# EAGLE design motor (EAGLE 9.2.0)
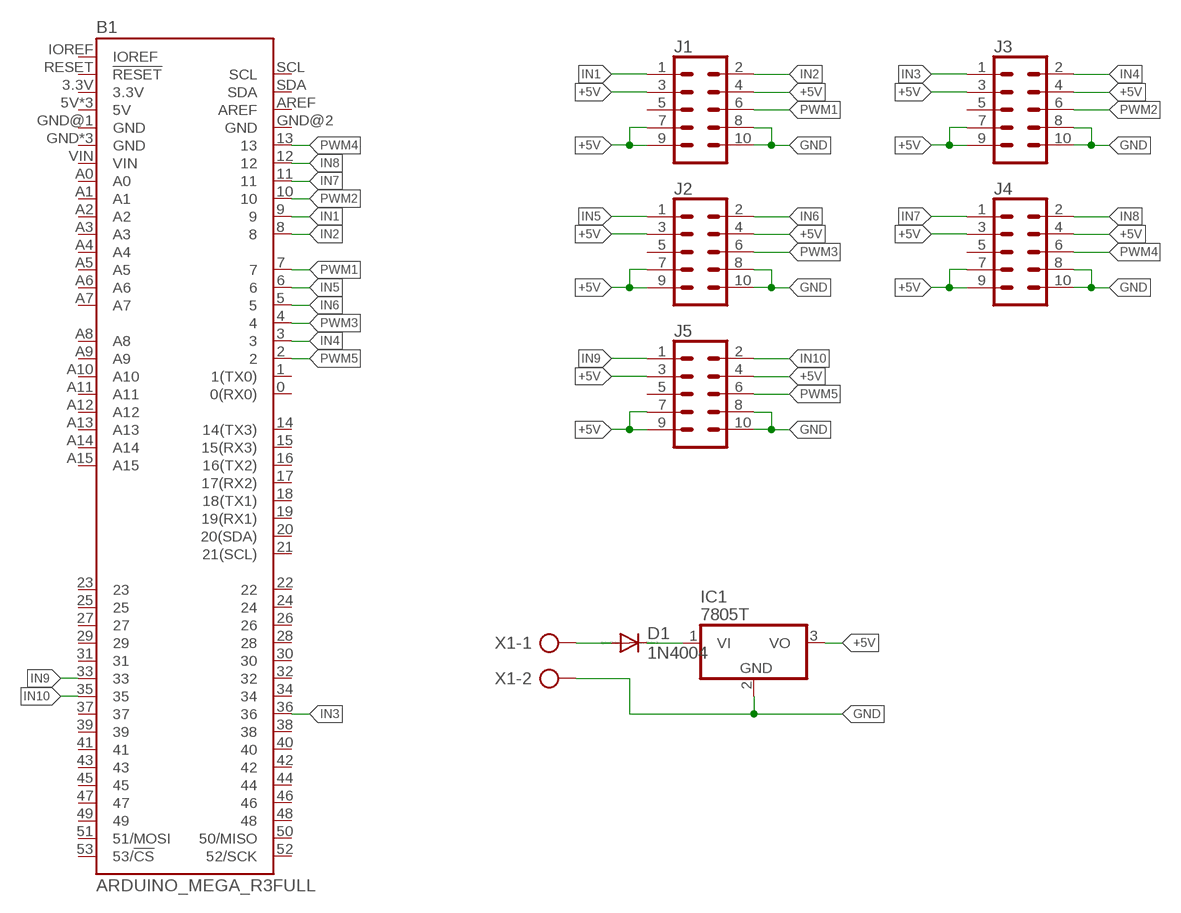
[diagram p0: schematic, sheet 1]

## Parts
B1  ARDUINO_MEGA_R3FULL  [ARDUINO_MEGA_NO_SILK]
D1  1N4004  [DO41-10]
IC1  7805T  [TO220H]
J1  CONN_05X2SHD-NS  [2X5-SHROUDED-NS]
J2  CONN_05X2SHD-NS  [2X5-SHROUDED-NS]
J3  CONN_05X2SHD-NS  [2X5-SHROUDED-NS]
J4  CONN_05X2SHD-NS  [2X5-SHROUDED-NS]
J5  CONN_05X2SHD-NS  [2X5-SHROUDED-NS]
X1  AK300/2  [AK300/2]

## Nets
+5V: IC1.3(VO) J1.3 J1.4 J1.7 J1.9 J2.3 J2.4 J2.7 J2.9 J3.3 J3.4 J3.7 J3.9 J4.3 J4.4 J4.7 J4.9 J5.3 J5.4 J5.7 J5.9
GND: IC1.2(GND) J1.8 J1.10 J2.8 J2.10 J3.8 J3.10 J4.8 J4.10 J5.8 J5.10 X1.2
IN1: B1.9 J1.1
IN2: B1.8 J1.2
IN3: B1.36 J3.1
IN4: B1.3 J3.2
IN5: B1.6 J2.1
IN6: B1.5 J2.2
IN7: B1.11 J4.1
IN8: B1.12 J4.2
IN9: B1.33 J5.1
IN10: B1.35 J5.2
N$1: D1.C IC1.1(VI)
N$2: D1.A X1.1
PWM1: B1.7 J1.6
PWM2: B1.10 J3.6
PWM3: B1.4 J2.6
PWM4: B1.13 J4.6
PWM5: B1.2 J5.6
Unconnected: B1.0(0(RX0)) B1.1(1(TX0)) B1.3.3V B1.5V B1.5V@1(5V) B1.5V@2(5V) B1.14(14(TX3)) B1.15(15(RX3)) B1.16(16(TX2)) B1.17(17(RX2)) B1.18(18(TX1)) B1.19(19(RX1)) B1.20(20(SDA)) B1.21(21(SCL)) B1.22 B1.23 B1.24 B1.25 B1.26 B1.27 B1.28 B1.29 B1.30 B1.31 B1.32 B1.34 B1.37 B1.38 B1.39 B1.40 B1.41 B1.42 B1.43 B1.44 B1.45 B1.46 B1.47 B1.48 B1.49 B1.50(50/MISO) B1.51(51/MOSI) B1.52(52/SCK) B1.53(53/!CS) B1.A0 B1.A1 B1.A2 B1.A3 B1.A4 B1.A5 B1.A6 B1.A7 B1.A8 B1.A9 B1.A10 B1.A11 B1.A12 B1.A13 B1.A14 B1.A15 B1.AREF B1.GND B1.GND@1(GND) B1.GND@2(GND) B1.GND@3(GND) B1.GND@4(GND) B1.IOREF B1.RESET(!RESET) B1.SCL B1.SDA B1.VIN J1.5 J2.5 J3.5 J4.5 J5.5

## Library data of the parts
B1 = SparkFun-Boards:ARDUINO_MEGA_R3: Arduino Mega R3 ATmega2560 R3 compatible footprint. SparkFun Products: Arduino Mega 2560 R3
D1 = diode:1N4004: DIODE
IC1 = linear:78*: Positive VOLTAGE REGULATOR Source: http://cache.national.com/ds/LM/LM78L05.pdf http://www.fairchildsemi.com/ds/LM/LM7805.pdf
J1-J5 = SparkFun-Connectors:CONN_05X2: Multi connection point. Often used as Generic Header-pin footprint for 0.1 inch spaced/style header connections For AVR SPI programming port, see special device with nice symbol: "AVR_SPI_PROG_5x2.dev" You can populate with any combo of single row headers, but if you'd like an exact match, check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; PROD_ID: CONN-08671; SF_ID: PRT-08506
X1 = con-ptr500:AK300/2: CONNECTOR; OC_FARNELL: unknown; OC_NEWARK: unknown

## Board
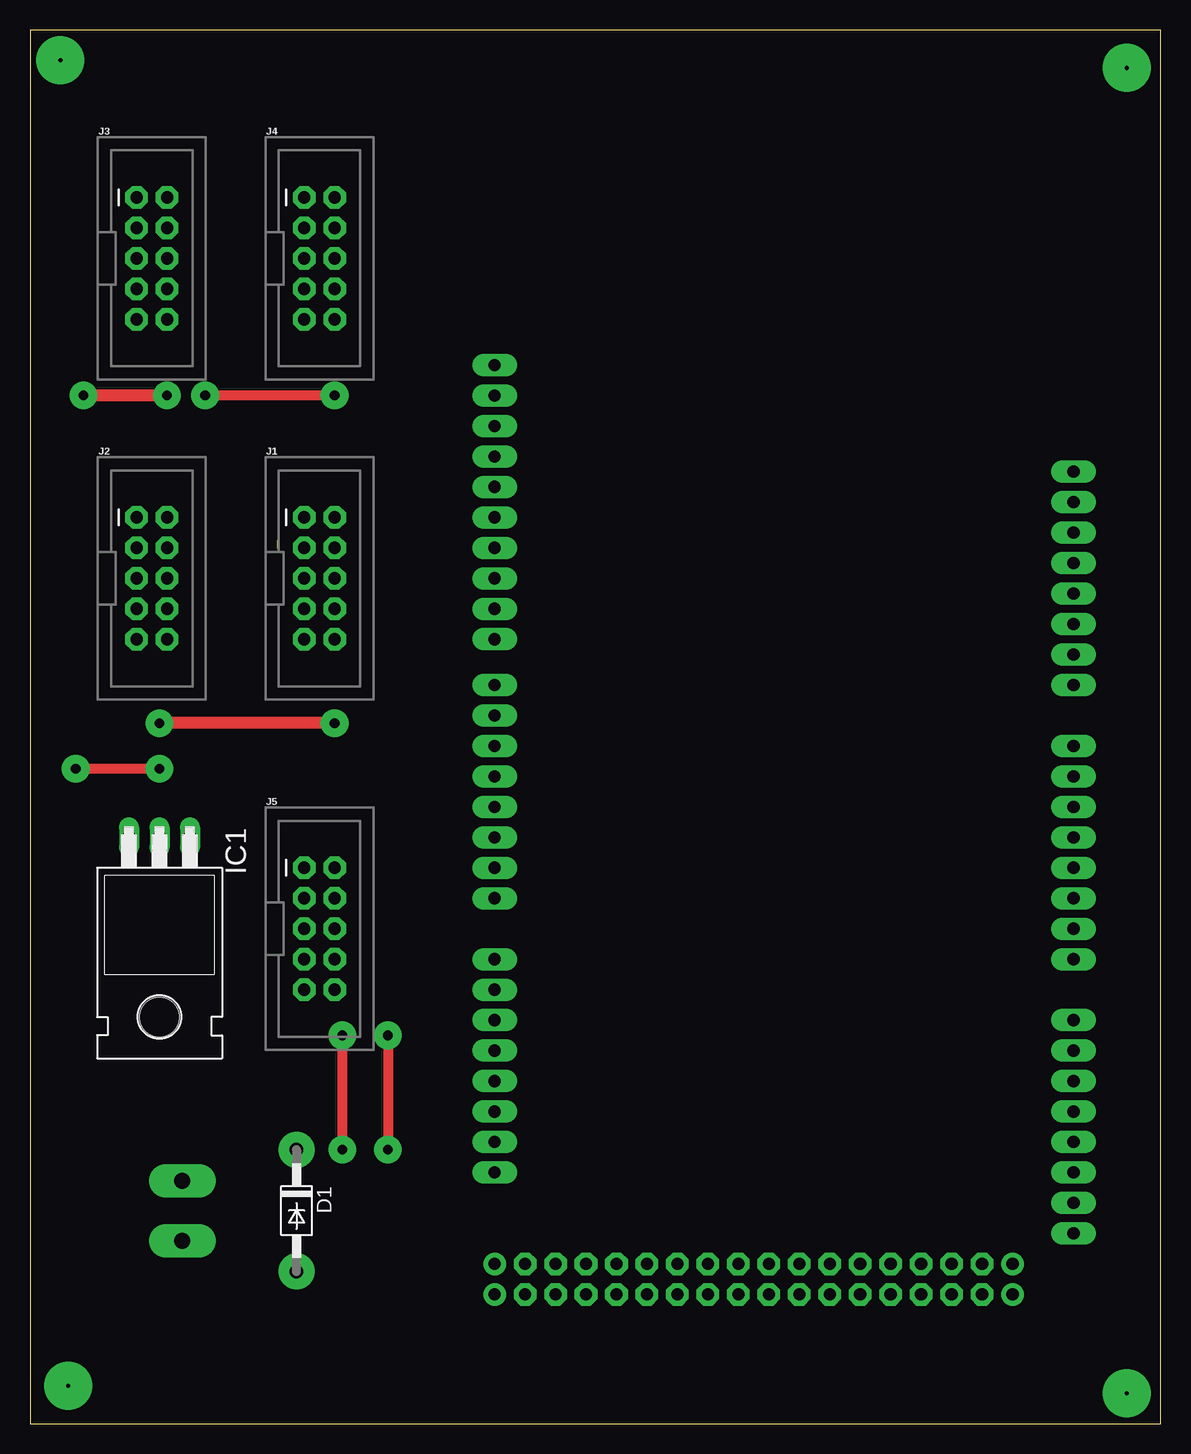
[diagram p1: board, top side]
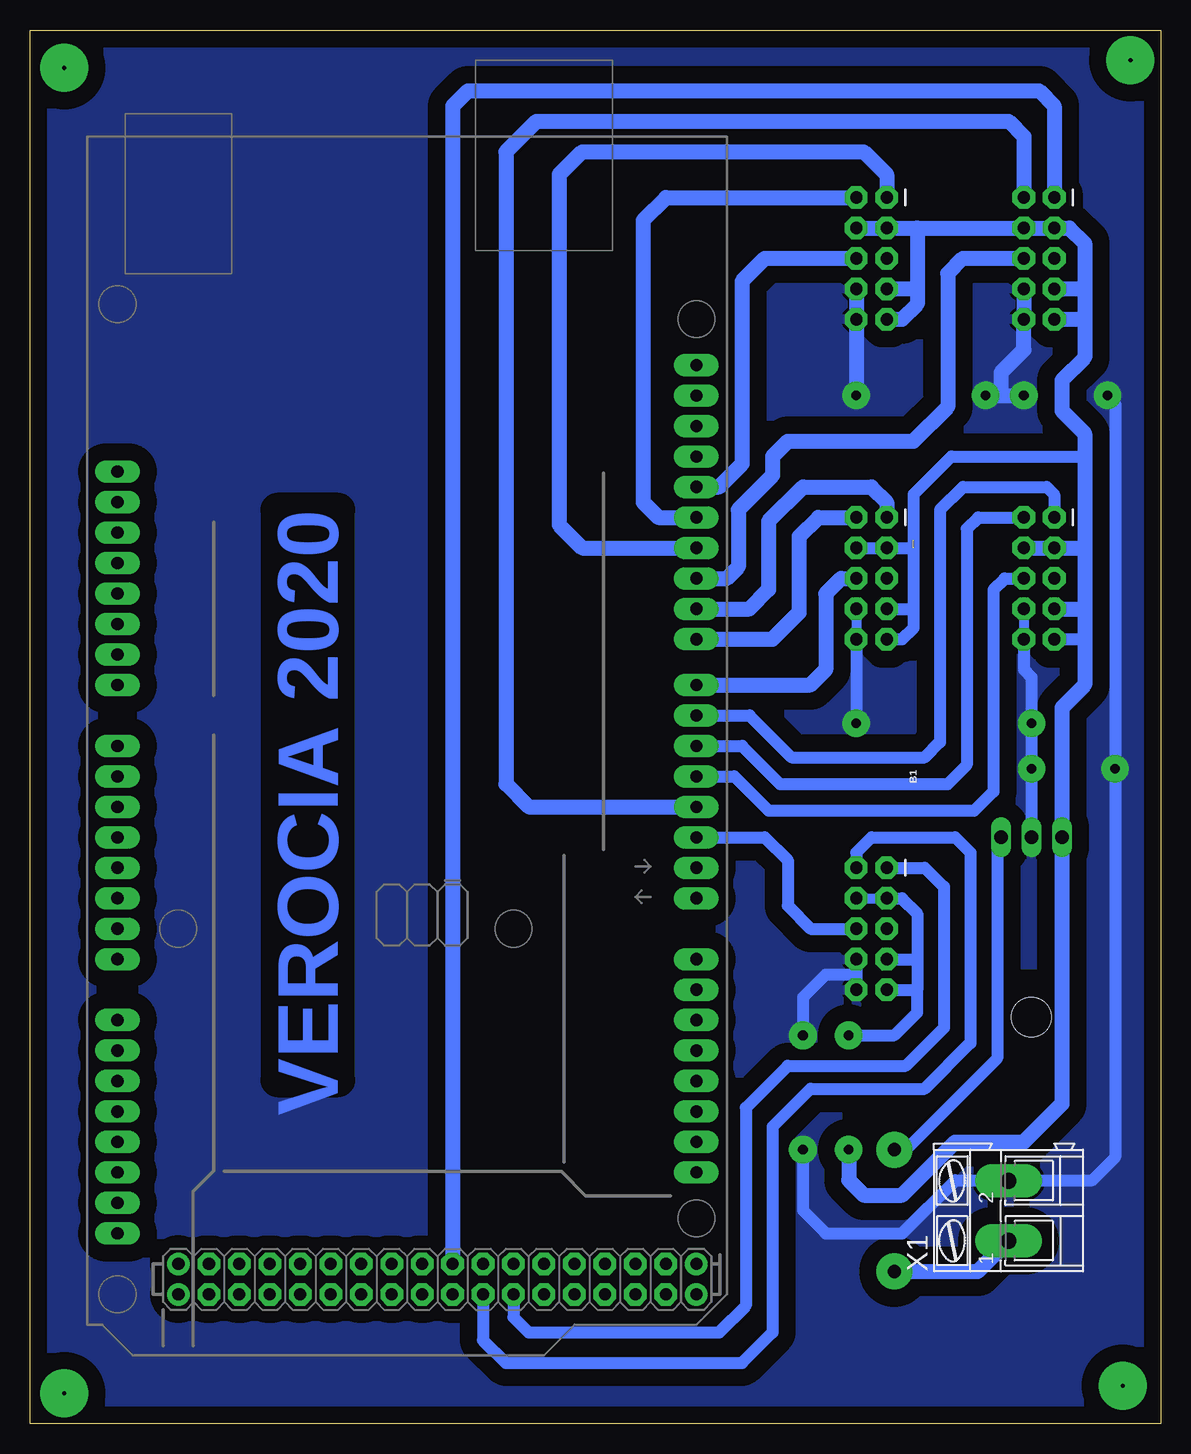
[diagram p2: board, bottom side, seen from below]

Size 94.28 x 116.19 mm. Coordinates in mm from the lower left corner, seen from the top.
Outline: 0,0 94.28,0 94.28,116.19 0,116.19 0,0
Copper layers (1*16): Top 0.035mm / dielectric 1.5mm / Bottom 0.035mm
Design rules "default": minimum track width 6mil, minimum drill 0.35mm, track to track 6mil, track to pad 6mil, pad to pad 6mil, via to via 6mil, smd to smd 6mil, copper to edge 40mil, drill to drill 6mil, minimum pad ring 10mil, minimum via ring 8mil, stop-mask expansion 4mil, vias tented up to drill 0mil, thermal gap 10mil

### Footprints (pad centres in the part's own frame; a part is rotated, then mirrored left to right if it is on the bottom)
ARDUINO_MEGA_NO_SILK = drill 1.016 pad 1.88 long: 0 13.97,24.13; 1 11.43,24.13; 2 8.89,24.13; 3 6.35,24.13; 3.3V -13.97,-24.13; 4 3.81,24.13; 5 1.27,24.13; 5V -11.43,-24.13; 6 -1.27,24.13; 7 -3.81,24.13; 8 -7.62,24.13; 9 -10.16,24.13; 10 -12.7,24.13; 11 -15.24,24.13; 12 -17.78,24.13; 13 -20.32,24.13; 14 19.05,24.13; 15 21.59,24.13; 16 24.13,24.13; 17 26.67,24.13; 18 29.21,24.13; 19 31.75,24.13; 20 34.29,24.13; 21 36.83,24.13; A0 1.27,-24.13; A1 3.81,-24.13; A2 6.35,-24.13; A3 8.89,-24.13; A4 11.43,-24.13; A5 13.97,-24.13; A6 16.51,-24.13; A7 19.05,-24.13; A8 24.13,-24.13; A9 26.67,-24.13; A10 29.21,-24.13; A11 31.75,-24.13; A12 34.29,-24.13; A13 36.83,-24.13; A14 39.37,-24.13; A15 41.91,-24.13; AREF -25.4,24.13; GND -8.89,-24.13; GND@1 -6.35,-24.13; GND@4 -22.86,24.13; IOREF -19.05,-24.13; NC -21.59,-24.13; RESET -16.51,-24.13; SCL -30.48,24.13; SDA -27.94,24.13; VIN -3.81,-24.13 | drill 1.016 pad 1.88: 5V@1 44.45,24.13; 5V@2 46.99,24.13; GND@2 44.45,-19.05; GND@3 46.99,-19.05 | drill 1.016 pad 1.88 octagon: 22 44.45,21.59; 23 46.99,21.59; 24 44.45,19.05; 25 46.99,19.05; 26 44.45,16.51; 27 46.99,16.51; 28 44.45,13.97; 29 46.99,13.97; 30 44.45,11.43; 31 46.99,11.43; 32 44.45,8.89; 33 46.99,8.89; 34 44.45,6.35; 35 46.99,6.35; 36 44.45,3.81; 37 46.99,3.81; 38 44.45,1.27; 39 46.99,1.27; 40 44.45,-1.27; 41 46.99,-1.27; 42 44.45,-3.81; 43 46.99,-3.81; 44 44.45,-6.35; 45 46.99,-6.35; 46 44.45,-8.89; 47 46.99,-8.89; 48 44.45,-11.43; 49 46.99,-11.43; 50 44.45,-13.97; 51 46.99,-13.97; 52 44.45,-16.51; 53 46.99,-16.51
DO41-10 = drill 1.118 pad 3: A 5.08,0; C -5.08,0
TO220H = drill 1.118 long: 1 -2.54,-10.16; 2 0,-10.16; 3 2.54,-10.16 | hole 3.302: 0,4.826
2X5-SHROUDED-NS = drill 1.016 pad 1.88 octagon: 1 -1.27,5.08; 2 1.27,5.08; 3 -1.27,2.54; 4 1.27,2.54; 5 -1.27,0; 6 1.27,0; 7 -1.27,-2.54; 8 1.27,-2.54; 9 -1.27,-5.08; 10 1.27,-5.08
AK300/2 = drill 1.321 pad 2.8 long: 1 -2.515,0; 2 2.489,0

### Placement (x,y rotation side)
B1  62.87,57.78 270 bottom
D1  22.23,17.78 270 top
IC1  10.79,38.73 180 top
J1  24.13,70.48 0 top
J2  10.16,70.48 0 top
J3  10.16,97.16 0 top
J4  24.13,97.16 0 top
J5  24.13,41.27 0 top
X1  12.7,17.78 90 bottom

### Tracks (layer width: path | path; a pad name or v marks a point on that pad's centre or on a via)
+5V  (via drill 0.8 pad 2.3)  (1 unrouted)
  Top 0.813: v26.04,32.38 v26.04,22.86
  Bottom 0.152: 20.32,39.05 20.32,38.73
  Bottom 0.813: J2.3 6.99,73.03 | J5.4 J5.3 | J4.3 20.32,99.69
  Bottom 1.016: J5.3 21.59,43.81 20.32,42.55 20.32,38.73 J5.7 | J5.9 20.32,36.2 | 20.32,39.05 20.32,36.2 | J1.4 J1.3 20.64,73.03 20.64,77.47 17.46,80.64 6.35,80.64 | 20.64,73.66 20.64,67.94 | 20.64,67.94 20.64,66.36 21.59,65.41 J1.9 | J1.7 20.64,67.94 | J2.9 6.35,65.41 | 20.32,36.2 20.32,34.29 22.23,32.38 v26.04,32.38
  Bottom 1.27: J2.4 J2.3 6.35,73.03 | J4.9 21.59,92.08 20.32,93.34 20.32,94.61 | 20.32,99.69 20.32,94.61 | J4.4 J4.3 J3.4 J3.3 7.62,99.69 6.35,98.42 6.35,94.61 | J4.7 20.32,94.61 | 6.35,67.94 6.35,65.41 6.35,61.59 8.26,59.69 IC1.3 8.26,26.67 11.43,23.5 17.14,23.5 21.59,19.05 24.77,19.05 26.04,20.32 v26.04,22.86 | J2.7 6.35,67.94 | 6.35,73.03 6.35,67.94 | 6.35,73.03 6.35,80.64 6.35,82.55 8.26,84.45 8.26,87 6.35,88.9 6.35,92.08 | 6.35,94.61 6.35,92.08 | J3.7 6.35,94.61 | J3.9 6.35,92.08
GND  (via drill 0.8 pad 2.3)
  Top 0.813: v25.4,85.72 v14.61,85.72 | v10.79,54.61 v3.81,54.61 | v29.84,32.38 v29.84,22.86
  Top 1.016: v11.43,85.72 v4.45,85.72 | v25.4,58.42 v10.79,58.42
  Bottom 0.813: J2.8 J2.10 | v14.61,85.72 13.34,85.72 | J1.8 J1.10
  Bottom 1.016: J5.8 25.4,37.47 | 25.4,37.47 J5.10 | IC1.2 v10.79,54.61 v10.79,58.42 10.79,62.23 11.43,62.87 J2.10 | X1.2 12.65,20.32 11.43,20.32 | v4.45,85.72 3.81,85.09 v3.81,54.61 3.81,22.23 5.71,20.32 11.43,20.32 | J1.10 v25.4,58.42 | v29.84,32.38 29.84,35.56 27.94,37.47 25.4,37.47 | v29.84,22.86 29.84,17.78 27.94,15.88 21.59,15.88 17.14,20.32 11.43,20.32
  Bottom 1.27: J4.8 J4.10 v25.4,85.72 | J3.8 J3.10 11.43,89.53 13.34,87.63 13.34,85.72 | v14.61,85.72 v11.43,85.72
  pour Bottom (isolate 1.422): 0,0 0,116.2 94.61,116.2 94.61,0
IN1
  Bottom 1.27: J1.1 22.86,76.83 24.13,78.11 29.84,78.11 32.7,75.25 32.7,69.53 34.29,67.94 B1.9
IN2
  Bottom 1.27: J1.2 28.57,75.56 30.16,73.98 30.16,67.63 32.38,65.41 B1.8
IN3
  Bottom 1.27: J3.1 8.89,109.86 10.16,111.12 57.78,111.12 59.05,109.86 B1.36
IN4
  Bottom 1.27: J3.2 11.43,107.31 12.7,108.58 52.07,108.58 54.61,106.05 54.61,53.34 52.7,51.44 B1.3
IN5
  Bottom 1.016: J2.1 8.89,77.47 9.53,78.11 16.51,78.11 18.41,76.2 18.41,56.83 19.68,55.56 30.8,55.56 34.29,59.05 B1.6
IN6
  Bottom 1.016: J2.2 15.24,75.56 16.19,74.61 16.19,54.93 17.78,53.34 31.75,53.34 34.92,56.52 B1.5
IN7
  Bottom 1.27: B1.11 48.26,73.03 50.16,74.93 50.16,104.14 48.26,106.05 24.77,106.05 22.86,104.14 J4.1
IN8
  Bottom 1.27: B1.12 41.91,75.56 43.18,76.83 43.18,100.33 41.27,102.23 J4.2
IN9
  Bottom 1.016: J5.1 19.68,46.35 18.1,44.77 18.1,33.02 21.27,29.84 31.11,29.84 34.61,26.35 34.61,9.84 36.83,7.62 52.7,7.62 53.98,8.89 B1.33
IN10
  Bottom 1.016: J5.2 25.4,47.62 24.13,48.9 17.14,48.9 15.88,47.62 15.88,31.75 19.68,27.94 29.21,27.94 32.38,24.77 32.38,7.62 34.92,5.08 54.61,5.08 56.52,6.99 B1.35
N$1
  Bottom 1.016: D1.C 21.27,22.86 13.65,30.48 13.65,48.58 IC1.1
N$2
  Bottom 1.27: X1.1 15.27,12.7 D1.A
N$3  (via drill 0.35 pad 4)
  other vias: 2.54,113.67
N$4  (via drill 0.35 pad 4)
  other vias: 91.44,113.03
N$5  (via drill 0.35 pad 4)
  other vias: 91.44,2.54
N$6  (via drill 0.35 pad 4)
  other vias: 3.17,3.17
PWM1
  Bottom 1.27: J1.6 26.67,70.48 27.94,69.22 27.94,62.87 29.21,61.59 B1.7
PWM2
  Bottom 1.27: J3.6 16.51,97.16 17.78,95.89 17.78,84.77 20.64,81.92 31.11,81.92 32.38,80.64 32.38,79.06 35.24,76.2 35.24,71.44 36.2,70.48 B1.10
PWM3
  Bottom 1.016: J2.6 13.02,70.48 13.97,69.53 13.97,52.7 15.56,51.12 32.7,51.12 35.56,53.98 B1.4
PWM4
  Bottom 1.27: J4.6 33.02,97.16 34.92,95.25 34.92,80.01 36.83,78.11 B1.13
PWM5
  Bottom 1.016: J5.6 29.21,41.27 31.11,43.18 31.11,46.99 33.02,48.9 B1.2

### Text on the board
Bottom: VEROCIA 2020

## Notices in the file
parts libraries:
SparkFun-Connectors: Licensing: Creative Commons ShareAlike 4.0 International - https://creativecommons.org/licenses/by-sa/4.0
